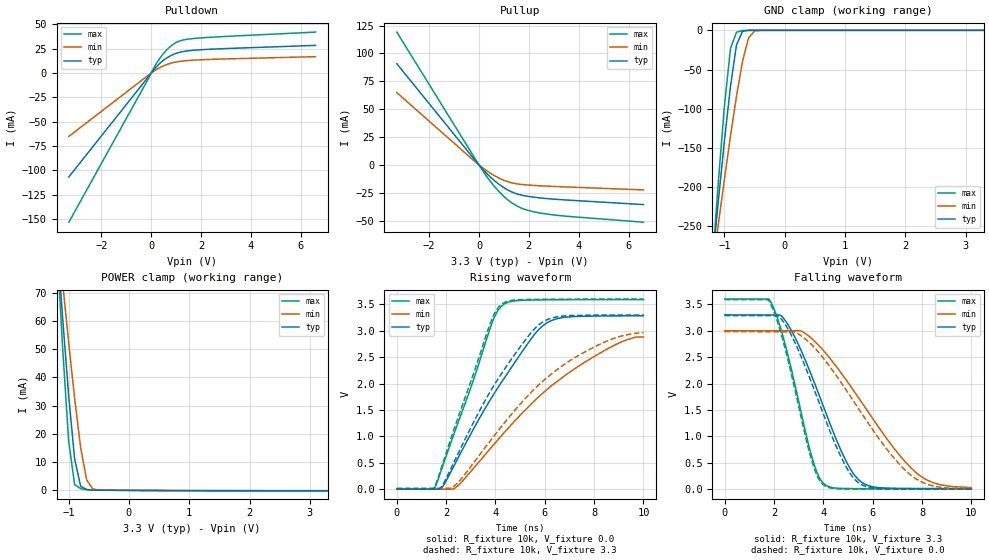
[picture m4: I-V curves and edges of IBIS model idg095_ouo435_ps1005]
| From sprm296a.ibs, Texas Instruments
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[Model]   idg095_ouo435_ps1005
Model_type   I/O
|  I/O with 100 UA pullup
Vinh = 2.00
Vinl = 0.80
Enable   Active-Low
Polarity   Non-Inverting
| signals   A, GZ, Y
Vmeas = 1.5
|   typ   min   max
C_comp   4.959p   4.901p   4.985p
|   typ   min   max
[Temperature Range]   25   -40   125
|   typ   min   max
[Voltage Range]   3.30V   3.00V   3.60V
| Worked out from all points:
|   slope of the pulldown table from 0 to 0.495 V, typ, clamps not added: 37.7 ohm
|   slope of the pullup table from 0 to 0.495 V, typ, clamps not added: 42.7 ohm
|   GND clamp passes 1 mA (typ) near -0.69 V on its own axis
|   POWER clamp passes 1 mA (typ) near -0.76 V on its own axis
|   rising waveform, R_fixture 10k, V_fixture 0.0: 20-80 % time 2.56ns typ, 3.85ns min, 1.59ns max; typ from 0 V to 3.28 V
|   falling waveform, R_fixture 10k, V_fixture 3.3: 20-80 % time 1.7ns typ, 2.74ns min, 1.09ns max; typ from 3.3 V to 0.011 V
|   rising waveform, R_fixture 10k, V_fixture 3.3: 20-80 % time 2.44ns typ, 3.55ns min, 1.57ns max; typ from 0.01 V to 3.3 V
|   falling waveform, R_fixture 10k, V_fixture 0.0: 20-80 % time 1.68ns typ, 2.69ns min, 1.09ns max; typ from 3.29 V to 0 V
[Pulldown]
|   Voltage   I(typ)   I(min)   I(max)
-3.3V     -106.6mA   -64.96mA   -153.1mA
-200mV    -6.638mA   -3.888mA   -9.861mA
200mV     6.136mA    3.487mA    9.379mA
500mV     13.23mA    7.514mA    20.3mA
800mV     18.12mA    10.25mA    27.98mA
1V        20.32mA    11.45mA    31.43mA
1.2V      21.76mA    12.24mA    33.52mA
1.7V      23.5mA     13.33mA    35.59mA
6.6V      28.52mA    16.93mA    42.18mA
[GND_clamp]
|   Voltage   I(typ)   I(min)   I(max)
-3.3V     -2.102A    -1.61A     -2.692A
-1.2V     -297mA     -305.4mA   -297.2mA
-1.1V     -217.4mA   -247.1mA   -192.9mA
-1V       -141.2mA   -190.1mA   -96.51mA
-900mV    -71.73mA   -135.3mA   -23.34mA
-800mV    -18.79mA   -84.08mA   -2.452mA
-700mV    -1.149mA   -39.68mA   -239uA
-600mV    -46.75uA   -9.694mA   -13.6uA
-500mV    -2.25uA    -862.3uA   -473.2nA
-300mV    -4.18nA    -2.906uA   -505.1pA
3.3V      222pA      386.7nA    310.9pA
[Pullup]
|   Voltage   I(typ)   I(min)   I(max)
-3.3V     90.83mA    64.92mA    119.1mA
100mV     -2.569mA   -1.78mA    -3.482mA
400mV     -9.588mA   -6.59mA    -13.07mA
700mV     -15.54mA   -10.57mA   -21.33mA
1.2V      -22.92mA   -15.27mA   -32mA
1.7V      -26.98mA   -17.44mA   -38.62mA
2V        -28.23mA   -18.01mA   -40.89mA
2.5V      -29.63mA   -18.7mA    -43.25mA
3.5V      -31.38mA   -19.67mA   -45.9mA
6.6V      -35.51mA   -22.36mA   -51.28mA
[POWER_clamp]
|   Voltage   I(typ)   I(min)   I(max)
-3.3V     767.3mA    589.7mA    982.7mA
-1.2V     90.9mA     95.6mA     89.15mA
-1.1V     61.46mA    73.73mA    50.93mA
-1V       33.86mA    52.55mA    17.61mA
-900mV    11.1mA     32.56mA    2.077mA
-800mV    1.423mA    15.1mA     614.5uA
-700mV    308.9uA    3.68mA     220.2uA
-600mV    110.7uA    509.4uA    114.4uA
-500mV    68.03uA    95.56uA    88.68uA
3.3V      -134.4uA   -85.9uA    -207.6uA
[Ramp]
|   I(typ)   I(min)   I(max)
dV/dt_r   1.970/2.558n   1.744/3.909n   2.154/1.590n
dV/dt_f   1.974/1.697n   1.782/2.736n   2.156/1.094n
[Rising Waveform]
R_fixture = 10k
V_fixture = 0.0
|  pu_on
|  TIME   V(typ)   V(min)   V(max)
0s        6nV        16nV       4nV
1.515ns   446uV      901.8uV    3.93nV
1.783ns   446uV      901.8uV    330.5mV
2.408ns   522.8mV    37.95mV    1.162V
3.926ns   1.795V     842.6mV    3.228V
4.373ns   2.114V     1.081V     3.511V
5.623ns   2.954V     1.692V     3.582V
6.249ns   3.189V     1.951V     3.586V
8.66ns    3.281V     2.688V     3.589V
10ns      3.284V     2.882V     3.59V
[Falling Waveform]
R_fixture = 10k
V_fixture = 3.3
V_fixture_min = 3.0
V_fixture_max = 3.6
|  pd_on
|  TIME   V(typ)   V(min)   V(max)
0s        3.3V       3V         3.6V
1.881ns   3.299V     2.998V     3.535V
2.299ns   3.283V     2.998V     2.999V
2.633ns   3.063V     2.998V     2.405V
3.552ns   2.114V     2.841V     578.9mV
4.053ns   1.504V     2.597V     88.05mV
4.972ns   485.4mV    2.035V     11.96mV
5.641ns   104mV      1.584V     9.3mV
7.896ns   13.05mV    262.6mV    7.352mV
10ns      10.78mV    30.6mV     7.076mV
[Rising Waveform]
R_fixture = 10k
V_fixture = 3.3
V_fixture_min = 3.0
V_fixture_max = 3.6
|  pd_off
|  TIME   V(typ)   V(min)   V(max)
0s        9.792mV    15.69mV    6.993mV
1.524ns   9.803mV    16.6mV     25.89mV
1.785ns   28.95mV    16.6mV     375.9mV
2.395ns   585.9mV    86.74mV    1.236V
3.789ns   1.849V     914.3mV    3.14V
4.224ns   2.172V     1.175V     3.492V
5.444ns   2.963V     1.833V     3.594V
6.054ns   3.201V     2.097V     3.596V
8.232ns   3.296V     2.744V     3.599V
10ns      3.298V     2.968V     3.6V
[Falling Waveform]
R_fixture = 10k
V_fixture = 0.0
|  pu_off
|  TIME   V(typ)   V(min)   V(max)
0s        3.287V     2.984V     3.59V
1.867ns   3.286V     2.982V     3.502V
2.193ns   3.273V     2.982V     3.09V
2.6ns     3.005V     2.982V     2.378V
3.497ns   2.044V     2.748V     590.7mV
3.985ns   1.44V      2.489V     87.87mV
4.882ns   456.2mV    1.907V     3.134mV
5.615ns   69.93mV    1.392V     1.177mV
7.733ns   1.137mV    201.3mV    178.7uV
10ns      282.1uV    4.705mV    38.34uV
